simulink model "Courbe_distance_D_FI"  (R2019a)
settings: Solver=VariableStepAuto  StartTime=0.0  StopTime=6.283185307  MaxStep=0.001  RelTol=1e-6  SampleTimeConstraint=STIndependent

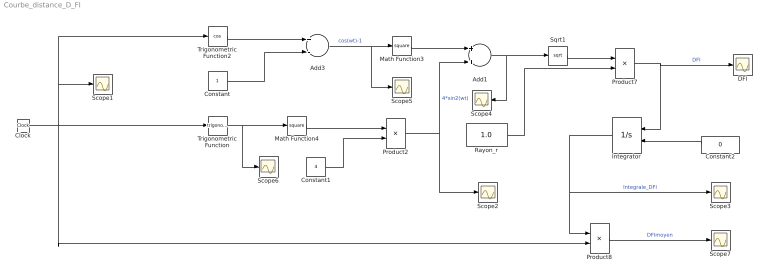
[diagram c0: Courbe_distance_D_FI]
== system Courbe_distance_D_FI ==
  Add1 : Sum
  Add3 : Sum  Inputs=+-
  Clock : Clock
  Constant : Constant
  Constant1 : Constant  Value=4
  Constant2 : Constant  Value=0
  DFI : Scope
  Integrator : Integrator  InitialConditionSource=external
  Math Function3 : Math  Operator=square
  Math Function4 : Math  Operator=square
  Product2 : Product
  Product7 : Product
  Product8 : Product  Inputs=*/
  Rayon_r : Constant  Value=1.0
  Scope{1..7} (7 alike) : Scope
  Sqrt1 : Sqrt
  Trigonometric Function : Trigonometry
  Trigonometric Function2 : Trigonometry  Operator=cos
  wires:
  Clock/1 -> Trigonometric Function/1, Trigonometric Function2/1, Scope1/1, Product8/2
  Integrator/1 -> Scope3/1, Product8/1  "Integrale_DFI"
  Constant2/1 -> Integrator/2
  Product8/1 -> Scope7/1  "DFImoyen"
  Trigonometric Function2/1 -> Add3/1
  Constant/1 -> Add3/2
  Add3/1 -> Scope5/1, Math Function3/1  "cos(wt)-1"
  Math Function3/1 -> Add1/1
  Trigonometric Function/1 -> Scope6/1, Math Function4/1
  Math Function4/1 -> Product2/1
  Constant1/1 -> Product2/2
  Product2/1 -> Scope2/1, Add1/2  "4*sin2(wt)"
  Add1/1 -> Scope4/1, Sqrt1/1
  Sqrt1/1 -> Product7/1
  Rayon_r/1 -> Product7/2
  Product7/1 -> DFI/1, Integrator/1  "DFI"
